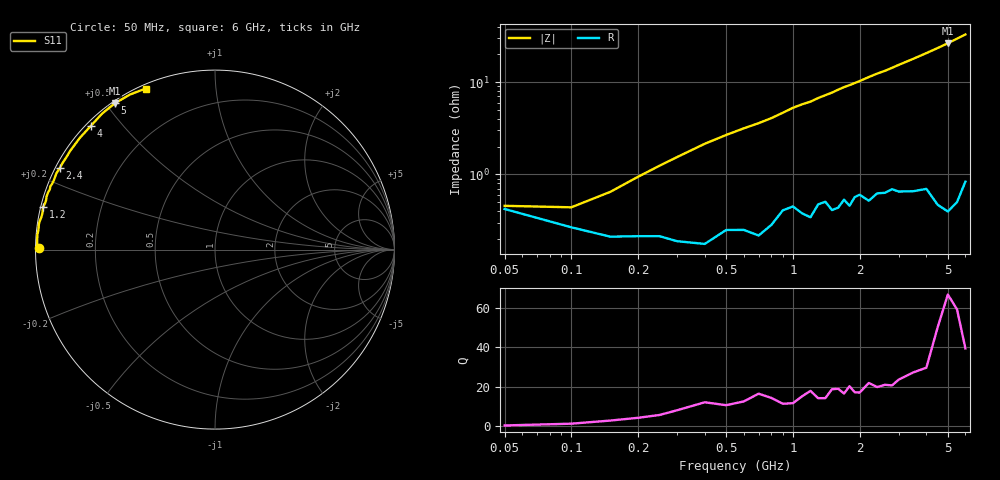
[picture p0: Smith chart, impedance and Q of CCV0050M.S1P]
! Infineon Technologies  Discrete & RF Semiconductors
! BBY57-02W
! Si Tuning Diode in SCD-80
! VR = 0
! S-Parameters:  June  2000
# GHz  S  MA  R  50
!  f  S11
! GHz  MAG  ANG
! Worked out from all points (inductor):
!   34 points, 50 MHz to 6 GHz, reference 50 ohm
!   read as one part to ground: L = 778 pH near 200 MHz
!   highest Q = 59.2 at 5 GHz (marker M1), where L = 841 pH
!   S11 on the Smith chart (normalised r, x): 50 MHz: 0.01, +0.00; 1.2 GHz: 0.01, +0.12; 2.4 GHz: 0.01, +0.25; 4 GHz: 0.01, +0.41; 5 GHz: 0.01, +0.53; 6 GHz: 0.02, +0.66
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0.05  0.9833 179.6
0.1  0.9894 179.2
0.15  0.9916 178.6
0.3  0.9925 176.5
0.4  0.993 175.1
0.5  0.9901 173.9
0.7  0.9914 171.8
0.8  0.9888 170.7
1  0.9824 168.0
1.1  0.9852 166.9
1.2  0.9866 166.0
1.3  0.9816 164.7
1.4  0.9804 163.6
1.5  0.9841 162.5
1.6  0.9832 161.2
1.7  0.9796 160.0
1.8  0.9825 159.0
2  0.9772 156.8
2.2  0.9805 154.4
2.4  0.9768 152.2
2.6  0.9767 150.3
3  0.9765 145.8
3.5  0.977 140.5
4  0.9765 135.1
4.5  0.9848 129.7
5  0.9877 124.3
5.5  0.9853 118.7
6  0.977 113.3
